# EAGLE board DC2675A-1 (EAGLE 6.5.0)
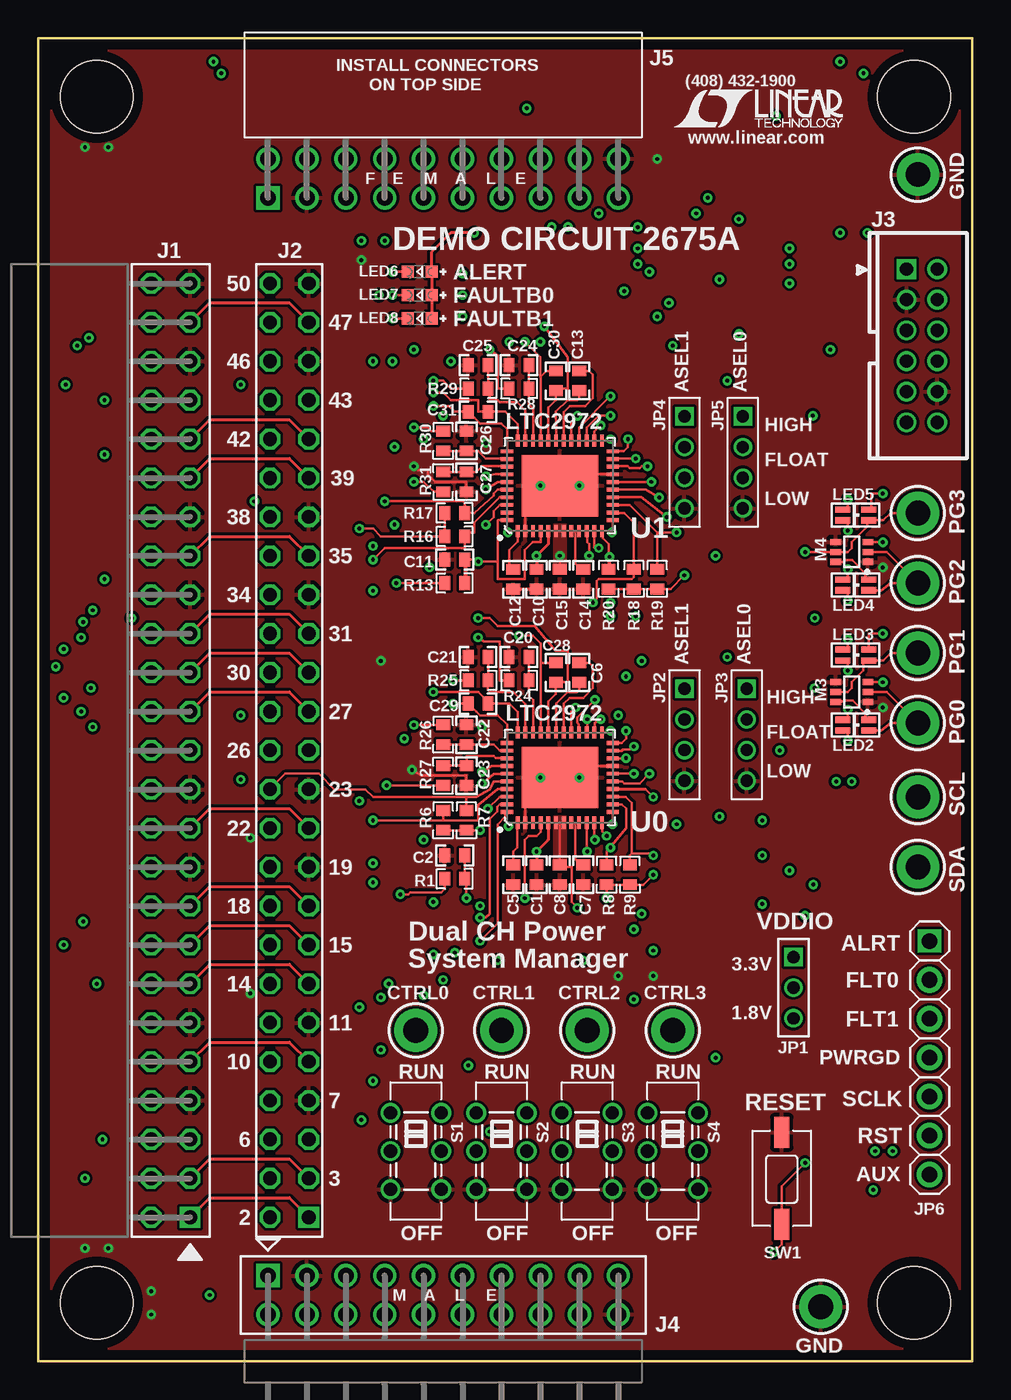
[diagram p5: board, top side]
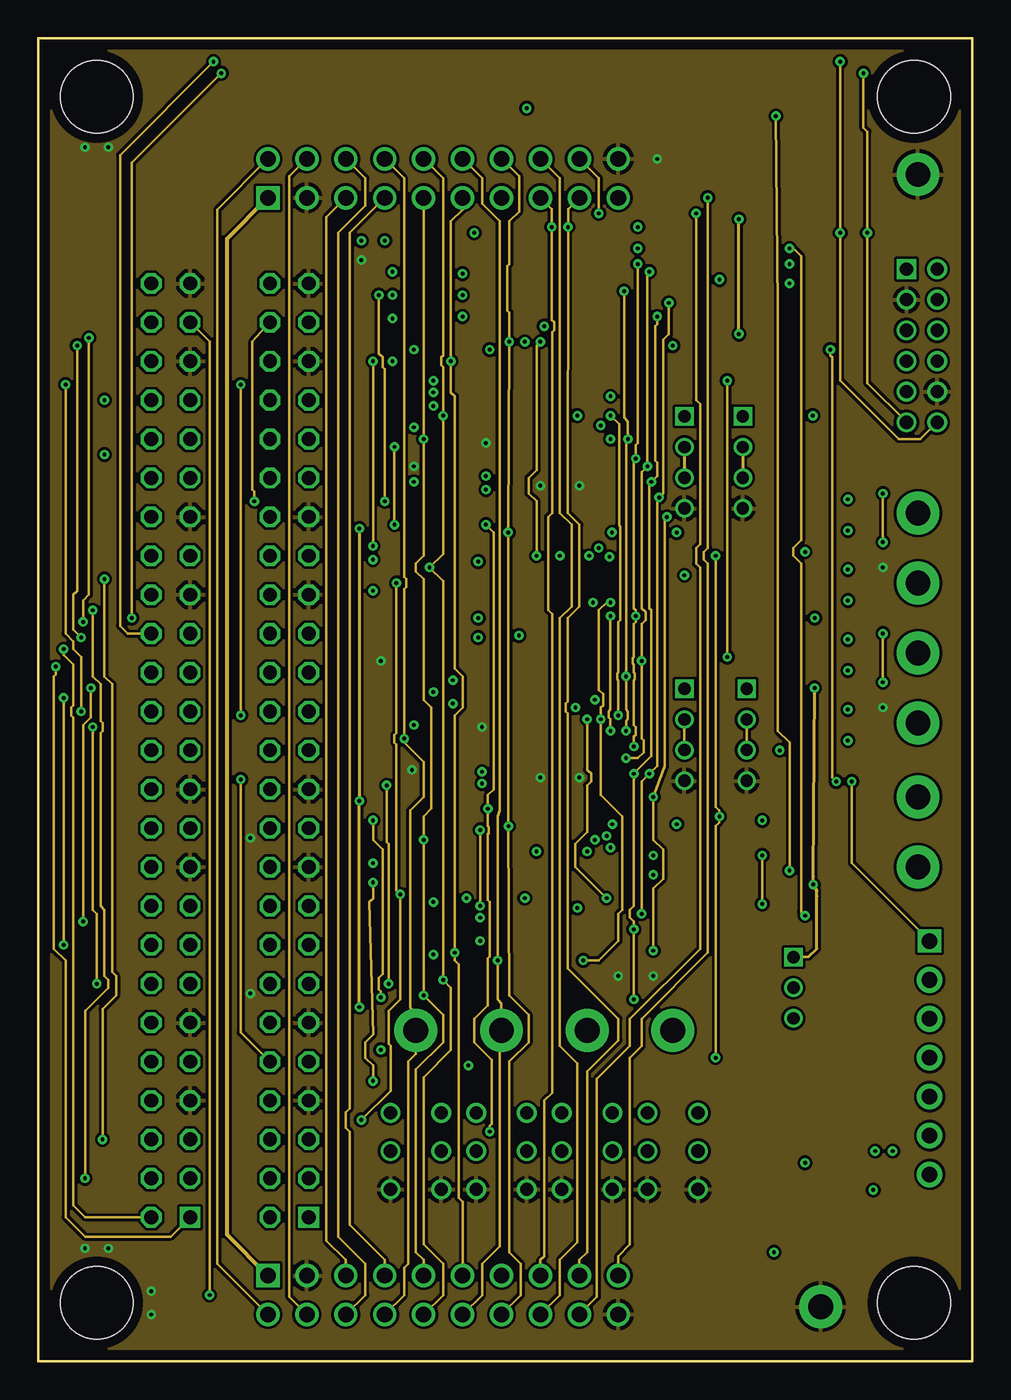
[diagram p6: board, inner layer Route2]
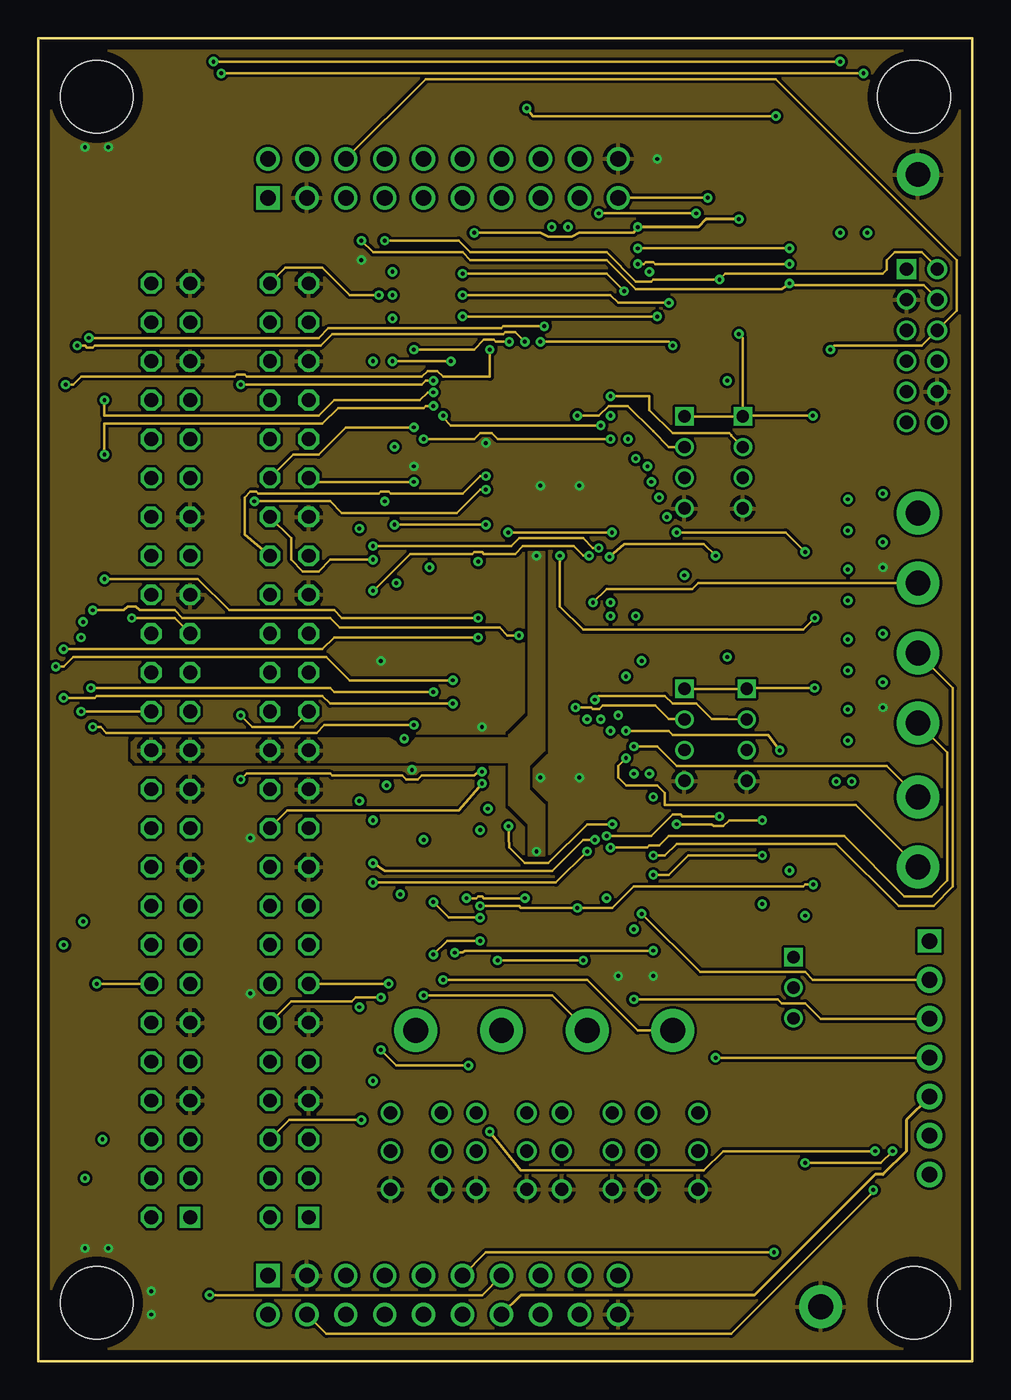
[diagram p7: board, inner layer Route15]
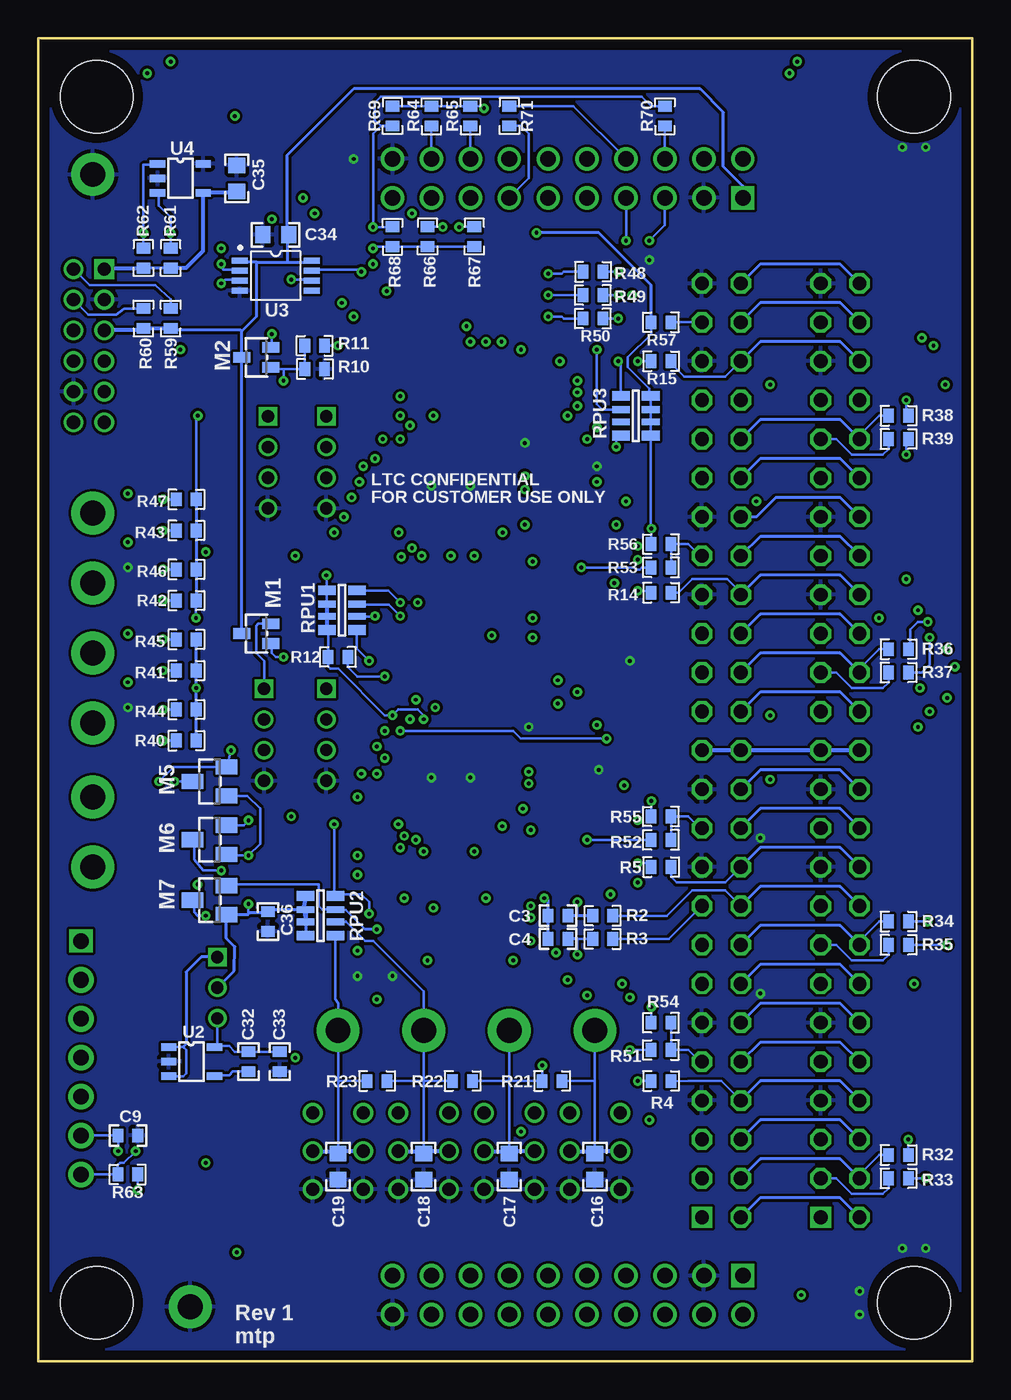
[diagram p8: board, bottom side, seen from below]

Size 60.96 x 86.36 mm. Coordinates in mm from the lower left corner, seen from the top.
Outline: 0,0 0,86.36 60.96,86.36 60.96,0 0.13,0
Copper layers (1*2+15*16): Top 0.07mm / dielectric 0.2mm / Route2 0.035mm / dielectric 1mm / Route15 0.035mm / dielectric 0.2mm / Bottom 0.07mm
Design rules "default *": minimum track width 6mil, minimum drill 10mil, track to track 6mil, track to pad 6mil, pad to pad 6mil, via to via 6mil, smd to smd 4mil, copper to edge 25mil, drill to drill 15mil, minimum pad ring 7mil, minimum via ring 7mil, stop-mask expansion 4mil, vias tented up to drill 15mil, thermal gap 10mil
Holes 4.75 mm at 3.81,3.81 3.81,82.55 57.15,82.55 57.15,3.81

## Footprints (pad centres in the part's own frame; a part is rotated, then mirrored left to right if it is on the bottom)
C0402_BOX = smd 0.7 x 0.9: 1 -0.65,0; 2 0.65,0
C0603_BOX = smd 1 x 1.1: 1 -0.85,0; 2 0.85,0
PINHEAD_2X25_RECEPT = drill 0.9 square: 1 1.27,-30.48 | drill 0.9 octagon: 2 -1.27,-30.48; 3 1.27,-27.94; 4 -1.27,-27.94; 5 1.27,-25.4; 6 -1.27,-25.4; 7 1.27,-22.86; 8 -1.27,-22.86; 9 1.27,-20.32; 10 -1.27,-20.32; 11 1.27,-17.78; 12 -1.27,-17.78; 13 1.27,-15.24; 14 -1.27,-15.24; 15 1.27,-12.7; 16 -1.27,-12.7; 17 1.27,-10.16; 18 -1.27,-10.16; 19 1.27,-7.62; 20 -1.27,-7.62; 21 1.27,-5.08; 22 -1.27,-5.08; 23 1.27,-2.54; 24 -1.27,-2.54; 25 1.27,0; 26 -1.27,0; 27 1.27,2.54; 28 -1.27,2.54; 29 1.27,5.08; 30 -1.27,5.08; 31 1.27,7.62; 32 -1.27,7.62; 33 1.27,10.16; 34 -1.27,10.16; 35 1.27,12.7; 36 -1.27,12.7; 37 1.27,15.24; 38 -1.27,15.24; 39 1.27,17.78; 40 -1.27,17.78; 41 1.27,20.32; 42 -1.27,20.32; 43 1.27,22.86; 44 -1.27,22.86; 45 1.27,25.4; 46 -1.27,25.4; 47 1.27,27.94; 48 -1.27,27.94; 49 1.27,30.48; 50 -1.27,30.48
PINHEAD_2X25_RECEPT_NO_SILK = drill 0.9 square: 1 1.27,-30.48 | drill 0.9 octagon: 2 -1.27,-30.48; 3 1.27,-27.94; 4 -1.27,-27.94; 5 1.27,-25.4; 6 -1.27,-25.4; 7 1.27,-22.86; 8 -1.27,-22.86; 9 1.27,-20.32; 10 -1.27,-20.32; 11 1.27,-17.78; 12 -1.27,-17.78; 13 1.27,-15.24; 14 -1.27,-15.24; 15 1.27,-12.7; 16 -1.27,-12.7; 17 1.27,-10.16; 18 -1.27,-10.16; 19 1.27,-7.62; 20 -1.27,-7.62; 21 1.27,-5.08; 22 -1.27,-5.08; 23 1.27,-2.54; 24 -1.27,-2.54; 25 1.27,0; 26 -1.27,0; 27 1.27,2.54; 28 -1.27,2.54; 29 1.27,5.08; 30 -1.27,5.08; 31 1.27,7.62; 32 -1.27,7.62; 33 1.27,10.16; 34 -1.27,10.16; 35 1.27,12.7; 36 -1.27,12.7; 37 1.27,15.24; 38 -1.27,15.24; 39 1.27,17.78; 40 -1.27,17.78; 41 1.27,20.32; 42 -1.27,20.32; 43 1.27,22.86; 44 -1.27,22.86; 45 1.27,25.4; 46 -1.27,25.4; 47 1.27,27.94; 48 -1.27,27.94; 49 1.27,30.48; 50 -1.27,30.48
CONN_DC1613 = drill 0.86 square: 1 -5,-1 | drill 0.86: 2 -5,1; 3 -3,-1; 4 -3,1; 5 -1,-1; 6 -1,1; 7 1,-1; 8 1,1; 9 3,-1; 10 3,1; 11 5,-1; 12 5,1
HEADER_2X10_0.1INCH = drill 1.016 square: P$1 1.27,11.43 | drill 1.016: P$2 -1.27,11.43; P$3 1.27,8.89; P$4 -1.27,8.89; P$5 1.27,6.35; P$6 -1.27,6.35; P$7 1.27,3.81; P$8 -1.27,3.81; P$9 1.27,1.27; P$10 -1.27,1.27; P$11 1.27,-1.27; P$12 -1.27,-1.27; P$13 1.27,-3.81; P$14 -1.27,-3.81; P$15 1.27,-6.35; P$16 -1.27,-6.35; P$17 1.27,-8.89; P$18 -1.27,-8.89; P$19 1.27,-11.43; P$20 -1.27,-11.43
RECEPT_2X10_0.1INCH = drill 1.016 square: P$1 -1.27,11.43 | drill 1.016: P$2 1.27,11.43; P$3 -1.27,8.89; P$4 1.27,8.89; P$5 -1.27,6.35; P$6 1.27,6.35; P$7 -1.27,3.81; P$8 1.27,3.81; P$9 -1.27,1.27; P$10 1.27,1.27; P$11 -1.27,-1.27; P$12 1.27,-1.27; P$13 -1.27,-3.81; P$14 1.27,-3.81; P$15 -1.27,-6.35; P$16 1.27,-6.35; P$17 -1.27,-8.89; P$18 1.27,-8.89; P$19 -1.27,-11.43; P$20 1.27,-11.43
1X03-2MM = drill 0.8 square: 1 -2,0 | drill 0.8: 2 0,0; 3 2,0
1X04-2MM = drill 0.8 square: 1 -3,0 | drill 0.8: 2 -1,0; 3 1,0; 4 3,0
1X07 = drill 1.016 square: 1 -7.62,0 | drill 1.016 pad 1.676: 2 -5.08,0; 3 -2.54,0; 4 0,0; 5 2.54,0; 6 5.08,0; 7 7.62,0
LED-DUAL_1.6X0.8MM = smd 1 x 0.4: 1 0.85,-0.35; 2 -0.85,-0.35; 3 0.85,0.35; 4 -0.85,0.35
CHIPLED_0603 = smd 0.8 x 0.8: N 0,0.78; P 0,-0.78
SOT323 = smd 0.7 x 1.1: 1 -0.65,-0.95; 2 0.65,-0.95; 3 0,0.95
SOT-363 = smd 0.7 x 0.4: 1 -1.05,0.65; 2 -1.05,0; 3 -1.05,-0.65; 4 1.05,-0.65; 5 1.05,0; 6 1.05,0.65
SOT23 = smd 1 x 1.4: 1 -0.95,-1.1; 2 0.95,-1.1; 3 0,1.1
R0402_BOX = smd 0.7 x 0.9: 1 -0.65,0; 2 0.65,0
R_VISHAY_CRA06S = smd 1.15 x 0.63: R1_1 -0.975,1.295; R1_2 0.975,1.295; R4_1 -0.975,-1.295; R4_2 0.975,-1.295 | smd 1.15 x 0.44: R2_1 -0.975,0.4; R2_2 0.975,0.4; R3_1 -0.975,-0.4; R3_2 0.975,-0.4
JS202011CQN = drill 0.86: 1 -2.5,1.65; 2 0,1.65; 3 2.5,1.65; 4 -2.5,-1.65; 5 0,-1.65; 6 2.5,-1.65
SWITCH_PTS635 = smd 2 x 1: SW1 -3,0; SW2 3,0
TURRET_SMALL_2308 = drill 1.626 pad 2.794: TP1 0,0
QFN44-6X7 = smd 0.8 x 0.25: 1 -2.95,2.75; 2 -2.95,2.25; 3 -2.95,1.75; 4 -2.95,1.25; 5 -2.95,0.75; 6 -2.95,0.25; 7 -2.95,-0.25; 8 -2.95,-0.75; 9 -2.95,-1.25; 10 -2.95,-1.75; 11 -2.95,-2.25; 12 -2.95,-2.75; 23 2.95,-2.75; 24 2.95,-2.25; 25 2.95,-1.75; 26 2.95,-1.25; 27 2.95,-0.75; 28 2.95,-0.25; 29 2.95,0.25; 30 2.95,0.75; 31 2.95,1.25; 32 2.95,1.75; 33 2.95,2.25; 34 2.95,2.75 | smd 0.25 x 0.8: 13 -2.25,-3.45; 14 -1.75,-3.45; 15 -1.25,-3.45; 16 -0.75,-3.45; 17 -0.25,-3.45; 18 0.25,-3.45; 19 0.75,-3.45; 20 1.25,-3.45; 21 1.75,-3.45; 22 2.25,-3.45; 35 2.25,3.45; 36 1.75,3.45; 37 1.25,3.45; 38 0.75,3.45; 39 0.25,3.45; 40 -0.25,3.45; 41 -0.75,3.45; 42 -1.25,3.45; 43 -1.75,3.45; 44 -2.25,3.45 | smd 4 x 5: 45 0,0
SOT-23-5 = smd 1 x 0.5: 1 -1.649,0.95; 2 -1.649,0; 3 -1.649,-0.95; 4 1.333,-0.95; 5 1.333,0.95
MSOP-8 = smd 0.406 x 1.016: 1 -0.975,-2.35; 2 -0.325,-2.35; 3 0.325,-2.35; 4 0.975,-2.35; 5 0.975,2.35; 6 0.325,2.35; 7 -0.325,2.35; 8 -0.975,2.35
SOT-23-5' = smd 1 x 0.5: 1 -1.491,0.95; 2 -1.491,0; 3 -1.491,-0.95; 4 1.491,-0.95; 5 1.491,0.95

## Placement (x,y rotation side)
C1  0.1uF/16V  [C0402_BOX]  32.51,31.75 270 top
C2  0.1uF/16V  [C0402_BOX]  27.18,33.02 0 top
C3  1uF/16V  [C0402_BOX]  27.05,29.08 0 bottom
C4  1uF/16V  [C0402_BOX]  27.05,27.56 0 bottom
C5  10nF  [C0402_BOX]  30.99,31.75 90 top
C6  0.1uF  [C0402_BOX]  35.31,44.96 270 top
C7  0.1uF  [C0402_BOX]  35.56,31.75 270 top
C8  0.1uF  [C0402_BOX]  34.04,31.75 270 top
C9  10n  [C0402_BOX]  55.12,14.73 180 bottom
C10  0.1uF/16V  [C0402_BOX]  32.51,51.05 270 top
C11  0.1uF/16V  [C0402_BOX]  27.18,52.32 0 top
C12  10nF  [C0402_BOX]  30.99,51.05 90 top
C13  0.1uF  [C0402_BOX]  35.31,64.01 270 top
C14  0.1uF  [C0402_BOX]  35.56,51.05 270 top
C15  0.1uF  [C0402_BOX]  34.04,51.05 270 top
C16  1uF  [C0603_BOX]  24.64,12.7 270 bottom
C17  1uF  [C0603_BOX]  30.23,12.7 270 bottom
C18  1uF  [C0603_BOX]  35.81,12.7 270 bottom
C19  1uF  [C0603_BOX]  41.4,12.7 270 bottom
C20  10n  [C0402_BOX]  31.37,45.97 180 top
C21  10n  [C0402_BOX]  28.7,45.97 180 top
C22  10n  [C0402_BOX]  27.94,40.89 90 top
C23  10n  [C0402_BOX]  27.94,38.23 270 top
C24  10n  [C0402_BOX]  31.37,65.02 180 top
C25  10n  [C0402_BOX]  28.7,65.02 180 top
C26  10n  [C0402_BOX]  27.94,60.07 90 top
C27  10n  [C0402_BOX]  27.94,57.4 270 top
C28  10n  [C0402_BOX]  33.78,44.96 90 top
C29  10n  [C0402_BOX]  28.7,42.93 180 top
C30  10n  [C0402_BOX]  33.78,64.01 90 top
C31  10n  [C0402_BOX]  28.7,61.98 180 top
C32  10nF  [C0402_BOX]  47.24,19.56 270 bottom
C33  4.7uF/10V  [C0402_BOX]  45.21,19.56 270 bottom
C34  1uF  [C0603_BOX]  45.47,73.53 180 bottom
C35  1uF  [C0603_BOX]  48.01,77.22 90 bottom
C36  0.1uF  [C0402_BOX]  45.97,28.7 270 bottom
DRILEGEND  [DRILEGEND]  not placed on the board
J1  CONN_2X25_RECEPT  [PINHEAD_2X25_RECEPT]  8.64,39.88 0 top
J2  CONN_2X25_RECEPT_NO_SILK  [PINHEAD_2X25_RECEPT_NO_SILK]  16.38,39.88 0 top
J3  CONN_DC1613  [CONN_DC1613]  57.66,66.29 270 top
J4  HEADER_CONN_2X10_0.1INCH  [HEADER_2X10_0.1INCH]  26.42,4.32 90 top
J5  RECEPT_CONN_2X10_0.1INCH  [RECEPT_2X10_0.1INCH]  26.42,77.22 90 top
JP1  [1X03-2MM]  49.28,24.38 270 top
JP2  [1X04-2MM]  42.16,40.89 270 top
JP3  [1X04-2MM]  46.23,40.89 270 top
JP4  [1X04-2MM]  42.16,58.67 270 top
JP5  [1X04-2MM]  45.97,58.67 270 top
JP6  [1X07]  58.17,19.81 270 top
LED2  Kingbright  [LED-DUAL_1.6X0.8MM]  53.34,41.53 180 top
LED3  Kingbright  [LED-DUAL_1.6X0.8MM]  53.34,46.1 180 top
LED4  Kingbright  [LED-DUAL_1.6X0.8MM]  53.34,50.67 180 top
LED5  Kingbright  [LED-DUAL_1.6X0.8MM]  53.34,55.24 180 top
LED6  RED  [CHIPLED_0603]  24.89,71.12 90 top
LED7  RED  [CHIPLED_0603]  24.89,69.6 90 top
LED8  RED  [CHIPLED_0603]  24.89,68.07 90 top
M1  NTS4173P  [SOT323]  46.74,47.5 90 bottom
M2  NTS4173P  [SOT323]  46.74,65.53 90 bottom
M3  [SOT-363]  53.09,43.69 180 top
M4  [SOT-363]  53.09,52.83 180 top
M5  BSS138  [SOT23]  49.78,37.85 90 bottom
M6  BSS138  [SOT23]  49.78,34.04 90 bottom
M7  BSS138  [SOT23]  49.78,30.1 90 bottom
R1  0  [R0402_BOX]  27.18,31.5 180 top
R2  0  [R0402_BOX]  24.13,29.08 180 bottom
R3  0  [R0402_BOX]  24.13,27.56 180 bottom
R4  0  [R0402_BOX]  20.32,18.29 0 bottom
R5  0  [R0402_BOX]  20.32,32.26 0 bottom
R6  10k  [R0402_BOX]  26.42,35.31 270 top
R7  10k  [R0402_BOX]  27.94,35.31 270 top
R8  10k  [R0402_BOX]  37.08,31.75 270 top
R9  10k  [R0402_BOX]  38.61,31.75 270 top
R10  150k  [R0402_BOX]  42.93,64.77 0 bottom
R11  49.9k  [R0402_BOX]  42.93,66.29 180 bottom
R12  10k  [R0402_BOX]  41.4,45.97 180 bottom
R13  0  [R0402_BOX]  27.18,50.8 180 top
R14  0  [R0402_BOX]  20.32,50.16 0 bottom
R15  0  [R0402_BOX]  20.32,65.28 0 bottom
R16  10k  [R0402_BOX]  27.18,53.85 180 top
R17  10k  [R0402_BOX]  27.18,55.37 180 top
R18  10k  [R0402_BOX]  38.86,51.05 270 top
R19  10k  [R0402_BOX]  40.39,51.05 270 top
R20  10k  [R0402_BOX]  37.21,51.05 270 top
R21  0  [R0402_BOX]  27.43,18.29 0 bottom
R22  0  [R0402_BOX]  33.27,18.29 0 bottom
R23  0  [R0402_BOX]  38.86,18.29 0 bottom
R24  0  [R0402_BOX]  31.37,44.45 0 top
R25  0  [R0402_BOX]  28.7,44.45 0 top
R26  0  [R0402_BOX]  26.42,40.89 270 top
R27  0  [R0402_BOX]  26.42,38.23 90 top
R28  0  [R0402_BOX]  31.37,63.5 0 top
R29  0  [R0402_BOX]  28.7,63.5 0 top
R30  0  [R0402_BOX]  26.42,60.07 270 top
R31  0  [R0402_BOX]  26.42,57.4 90 top
R32  0  [R0402_BOX]  4.83,13.46 0 bottom
R33  0  [R0402_BOX]  4.83,11.94 0 bottom
R34  0  [R0402_BOX]  4.83,28.7 0 bottom
R35  0  [R0402_BOX]  4.83,27.18 0 bottom
R36  0  [R0402_BOX]  4.83,46.48 0 bottom
R37  0  [R0402_BOX]  4.83,44.96 0 bottom
R38  0  [R0402_BOX]  4.83,61.72 0 bottom
R39  0  [R0402_BOX]  4.83,60.2 0 bottom
R40  1.4k  [R0402_BOX]  51.31,40.51 0 bottom
R41  1.4k  [R0402_BOX]  51.31,45.09 0 bottom
R42  1.4k  [R0402_BOX]  51.31,49.66 0 bottom
R43  1.4k  [R0402_BOX]  51.31,54.23 0 bottom
R44  4k  [R0402_BOX]  51.31,42.55 0 bottom
R45  4k  [R0402_BOX]  51.31,47.12 0 bottom
R46  4k  [R0402_BOX]  51.31,51.69 0 bottom
R47  4k  [R0402_BOX]  51.31,56.26 0 bottom
R48  866  [R0402_BOX]  24.77,71.12 0 bottom
R49  866  [R0402_BOX]  24.77,69.6 180 bottom
R50  866  [R0402_BOX]  24.77,68.07 180 bottom
R51  0  [R0402_BOX]  20.32,20.32 180 bottom
R52  0  [R0402_BOX]  20.32,34.04 180 bottom
R53  0  [R0402_BOX]  20.32,51.82 180 bottom
R54  10k  [R0402_BOX]  20.32,22.1 180 bottom
R55  10k  [R0402_BOX]  20.32,35.56 180 bottom
R56  10k  [R0402_BOX]  20.32,53.34 180 bottom
R57  10k  [R0402_BOX]  20.32,67.82 180 bottom
R59  10k  [R0402_BOX]  52.32,68.07 90 bottom
R60  10k  [R0402_BOX]  54.1,68.07 90 bottom
R61  10k  [R0402_BOX]  52.32,72.01 270 bottom
R62  10k  [R0402_BOX]  54.1,72.01 270 bottom
R63  0 (DNI)  [R0402_BOX]  55.12,12.19 180 bottom
R64  0  [R0402_BOX]  35.31,81.28 90 bottom
R65  0  [R0402_BOX]  32.77,81.28 90 bottom
R66  0  [R0402_BOX]  35.56,73.41 270 bottom
R67  0  [R0402_BOX]  32.51,73.41 270 bottom
R68  10k  [R0402_BOX]  37.85,73.41 90 bottom
R69  10k  [R0402_BOX]  37.85,81.28 270 bottom
R70  10k  [R0402_BOX]  20.07,81.28 90 bottom
R71  0 (DNI)  [R0402_BOX]  30.23,81.28 270 bottom
RPU1  10k, 4X  [R_VISHAY_CRA06S]  41.15,49.02 180 bottom
RPU2  10k, 4X  [R_VISHAY_CRA06S]  42.55,29.08 180 bottom
RPU3  10k, 4X  [R_VISHAY_CRA06S]  21.97,61.72 0 bottom
S1  CONTROL0  [JS202011CQN]  24.64,13.72 270 top
S2  CONTROL1  [JS202011CQN]  30.23,13.72 270 top
S3  CONTROL2  [JS202011CQN]  35.81,13.72 270 top
S4  CONTROL3  [JS202011CQN]  41.4,13.72 270 top
SW1  PTS635SL25SMTR LFS  [SWITCH_PTS635]  48.51,11.94 90 top
TP1  [TURRET_SMALL_2308]  57.4,36.83 0 top
TP2  [TURRET_SMALL_2308]  57.4,32.26 0 top
TP3  [TURRET_SMALL_2308]  57.4,41.66 0 top
TP4  [TURRET_SMALL_2308]  57.4,46.23 0 top
TP5  [TURRET_SMALL_2308]  57.4,50.8 0 top
TP6  [TURRET_SMALL_2308]  57.4,55.37 0 top
TP7  [TURRET_SMALL_2308]  24.64,21.59 0 top
TP8  [TURRET_SMALL_2308]  30.23,21.59 0 top
TP9  [TURRET_SMALL_2308]  35.81,21.59 0 top
TP10  [TURRET_SMALL_2308]  41.4,21.59 0 top
TP11  [TURRET_SMALL_2308]  57.4,77.47 0 top
TP12  [TURRET_SMALL_2308]  51.05,3.56 0 top
U0  LTC2972  [QFN44-6X7]  34.04,38.1 90 top
U1  LTC2972  [QFN44-6X7]  34.04,57.15 90 top
U2  LT1761-1.8V  [SOT-23-5]  50.8,19.56 0 bottom
U3  LTC4313-3  [MSOP-8]  45.47,70.87 270 bottom
U4  24AA02T-I/OT  [SOT-23-5']  51.69,77.22 0 bottom
U$6  [DC2675_FRAME]  not placed on the board
U$86  [LT_LOGO_SILK_450MILS]  41.4,80.52 0 top

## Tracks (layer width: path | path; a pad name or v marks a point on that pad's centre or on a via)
1V8
  Bottom 0.152: C33.1 C32.1 48.15,20.21 48.51,20.57 49.4,20.57 U2.5 49.28,20.7 JP1.3
ALERTB  (via drill 0.25)
  Top 0.152: U1.22 38.19,59.4 38.48,59.69 v38.48,60.2 | U0.22 38.06,40.35 38.35,40.64 v38.35,41.15
  Route2 0.152: v38.23,69.85 38.23,61.59 38.48,61.34 v38.48,60.2 38.35,59.94 v38.35,44.7 38.35,42.55 38.48,42.42 38.48,41.91 38.35,41.78 v38.35,41.15 | v53.09,37.85 53.09,32.51 JP6.1
  Route15 0.152: v38.23,69.85 37.08,70.99 v27.69,70.99 | v38.35,41.15 41.15,41.15 41.4,40.89 47.62,40.89 v48.39,39.88
  Bottom 0.152: R12.1 40.75,45.32 40.13,44.7 v38.35,44.7 | v48.39,39.88 48.64,38.84 M5.2 52.14,38.8 v53.09,37.85 | R48.1 26.67,71.12 26.8,70.99 v27.69,70.99
ALERTB_3V3  (via drill 0.25)
  Route2 0.152: J4.P$6 21.34,4.32 21.34,6.35 19.56,8.13 19.56,73.66 21.34,75.44 21.34,77.22 J5.P$6 | v51.69,66.04 51.69,65.66 51.82,65.53 51.82,38.1 v52.07,37.85
  Route15 0.152: J5.P$6 25.27,83.69 48.13,83.69 59.94,71.88 59.94,68.58 J3.6 57.66,66.29 51.94,66.29 v51.69,66.04
  Bottom 0.152: R70.1 J5.P$6 | v52.07,37.85 M5.3
ASEL0_U0  (via drill 0.25)
  Top 0.152: U0.26 35.28,41.58 35.18,41.68 35.18,42.04 v36.32,43.18
  Route2 0.152: JP3.2 JP3.3
  Route15 0.152: v36.32,43.18 36.58,43.43 40.89,43.43 41.4,42.93 42.93,42.93 43.94,41.91 44.94,41.91 JP3.2
ASEL0_U1  (via drill 0.25)
  Top 0.152: U1.26 35.29,60.94 v37.34,62.99
  Route2 0.203: JP5.2 JP5.3
  Route15 0.152: v37.34,62.99 39.88,62.99 39.88,62.1 41.4,60.58 45.09,60.58 45.21,60.45 45.21,60.44 JP5.2
ASEL1_U0  (via drill 0.25)
  Top 0.152: U0.27 34.79,42.41 v35.05,42.67
  Route2 0.152: JP2.2 JP2.3
  Route15 0.152: v35.05,42.67 36.07,42.67 36.17,42.57 36.6,42.57 36.83,42.8 40.26,42.8 41.15,41.91 42.15,41.91 JP2.2
ASEL1_U1  (via drill 0.25)
  Top 0.152: U1.27 34.79,61.33 v35.18,61.72
  Route2 0.203: JP4.2 JP4.3
  Route15 0.152: v35.18,61.72 36.58,61.72 37.21,62.36 38.48,62.36 40.13,60.71 41.15,59.67 JP4.2
AUX_SCL  (via drill 0.25)
  Top 0.203: J1.31 11.18,48.77 16.38,48.77 J2.31
  Route2 0.152: J3.11 54.1,63.85 v54.1,73.66 54.1,80.26 53.85,80.52 v53.85,84.07 | v11.94,84.07 6.1,78.23 v6.1,48.51
  Route15 0.152: v53.85,84.07 v11.94,84.07 | v6.1,48.51 8.89,48.51 J1.31
  Bottom 0.152: U4.1 53.24,78.11 54.1,78.11 v54.1,73.66 R62.1
AUX_SDA  (via drill 0.25)
  Route2 0.152: J3.12 57.56,60.2 56.13,60.2 52.32,64.01 v52.32,73.66 v52.32,84.84 | v11.43,84.84 5.33,78.74 5.33,48.01 5.84,47.5 J1.32
  Route15 0.152: v52.32,84.84 v11.43,84.84
  Bottom 0.152: U4.3 53.09,76.17 53.09,75.44 52.32,74.68 v52.32,73.66 R61.1
  Bottom 0.203: J1.32 8.64,48.77 13.84,48.77 J2.32
AUXFAULTB  (via drill 0.25)
  Top 0.152: U0.42 30.57,36.83 30.1,36.83 v29.34,36.07 | U1.42 30.12,55.9 29.72,55.5 29.72,55.12 v29.21,54.61
  Route2 0.152: v29.46,14.99 29.46,15.37 29.59,15.49 29.59,19.68 28.45,20.83 28.45,22.35 29.34,23.24 29.34,26.29 29.46,26.42 29.46,29.97 29.34,30.1 29.34,34.42 29.39,34.47 29.39,34.87 29.34,34.92 v29.34,36.07 29.34,36.96 29.72,37.34 29.72,54.1 v29.21,54.61 | v23.24,54.61 v23.24,59.69
  Route15 0.152: v54.61,13.72 44.7,13.72 43.43,12.45 31.5,12.45 v29.46,14.99 | v29.21,54.61 v23.24,54.61
  Bottom 0.152: JP6.7 R63.2 55.77,12.81 55.63,12.95 55.37,12.95 v54.61,13.72 | v23.24,59.69 23.24,60.13 RPU3.R4_1
AUXFAULTB_3V3  (via drill 0.25)
  Route2 0.152: J4.P$4 16.38,4.19 16.38,77.34 J5.P$4
  Route15 0.152: v54.48,11.18 54.48,11.05 45.21,1.78 18.8,1.78 J4.P$4
  Bottom 0.152: R63.1 54.47,11.19 v54.48,11.18
CTRL0  (via drill 0.25)
  Top 0.152: U0.23 37.24,41.05 v37.34,41.15
  Route2 0.152: J4.P$8 23.88,4.32 23.88,6.1 24.13,6.35 24.13,19.56 24.64,20.07 TP7.TP1 24.64,22.35 24.26,23.11 24.26,35.94 25.15,36.83 25.15,39.12 23.88,40.39 v23.88,40.64 23.88,50.42 24,50.55 24,51.05 23.88,51.18 23.88,77.22 J5.P$8 | v37.34,41.15 37.34,41.91 37.24,42.04 37.24,42.42 37.34,42.55 v37.34,48.64
  Bottom 0.152: R21.2 24.64,18.29 | 24.64,18.29 C16.1 | 24.64,18.29 TP7.TP1 | v37.34,41.15 29.97,41.15 29.46,40.64 v23.88,40.64 | v37.34,48.64 38.1,49.4 40.15,49.4 RPU1.R3_1 | R71.1 26.05,81.93 J5.P$8
  Bottom 0.254: S1.5 24.64,13.72 | S1.2 24.64,13.72 | 24.64,13.72 C16.1
CTRL1  (via drill 0.25)
  Top 0.152: 36.32,41.4 36.32,41.09 U0.24 36.29,41.37 36.32,41.4 | 36.32,41.4 36.32,41.66 v36.7,41.91
  Route2 0.152: J4.P$12 28.96,4.32 28.96,6.35 30.1,7.49 30.1,20.07 30.23,21.08 TP8.TP1 30.23,23.37 29.97,23.62 v29.97,26.16 29.97,35.56 30.1,35.94 30.1,74.42 28.96,75.56 28.96,77.22 J5.P$12 | v37.34,49.53 37.08,49.53 36.58,49.02 36.58,43.81 36.85,43.56 36.85,42.8 36.7,42.67 v36.7,41.91 36.7,36.96 38.1,35.56 38.1,29.46 37.85,29.21 37.85,27.43 36.58,26.16 v35.56,26.16
  Route15 0.152: v22.35,20.32 23.37,19.3 v28.07,19.3 | v35.56,26.16 v29.97,26.16
  Bottom 0.152: 30.23,18.29 R21.1 28.07,18.3 v28.07,19.3 | 30.23,18.29 C17.1 | R22.2 30.23,18.29 | 30.23,18.29 TP8.TP1 | RPU1.R4_1 38.12,50.32 v37.34,49.53 | R51.2 v22.35,20.32
  Bottom 0.254: S2.5 30.23,13.72 | S2.2 30.23,13.72 | 30.23,13.72 C17.1
CTRL2  (via drill 0.25)
  Top 0.152: U1.23 37.24,60.1 v37.34,60.2
  Route2 0.152: J4.P$9 25.15,6.6 24.64,7.11 24.64,19.05 26.42,20.83 26.42,22.61 v25.15,23.88 v25.15,34.04 25.15,35.56 25.65,36.07 25.65,42.67 25.15,43.18 25.15,51.05 24.64,51.56 24.64,52.07 25.15,52.58 v25.15,60.2 J5.P$9
  Route15 0.152: v37.34,60.2 29.97,60.2 29.59,60.58 28.83,60.58 28.45,60.2 v25.15,60.2 | TP9.TP1 33.53,23.88 v25.15,23.88
  Bottom 0.152: R22.1 35.81,18.29 | 35.81,18.29 C18.1 | R23.2 35.81,18.29 | 35.81,18.29 TP9.TP1 35.81,24.13 39.12,27.43 39.62,27.43 40.89,28.7 40.91,28.68 RPU2.R2_1 | R52.2 v25.15,34.04
  Bottom 0.254: S3.5 35.81,13.72 | S3.2 35.81,13.72 | 35.81,13.72 C18.1
CTRL3  (via drill 0.25)
  Top 0.152: U1.24 36.29,60.67 v36.7,61.09
  Route2 0.152: J5.P$10 26.42,77.22 26.42,65.66 26.29,65.53 26.29,65.02 26.42,64.9 v26.42,61.72 26.42,52.7 v25.53,51.82 26.42,50.93 v26.42,24.89 26.92,24.38 26.92,20.32 25.15,18.54 25.15,7.62 26.42,6.35 26.42,4.32 J4.P$10
  Route15 0.152: v36.7,61.09 26.92,61.09 26.42,61.59 v26.42,61.72 | TP10.TP1 39.12,21.59 35.81,24.89 v26.42,24.89
  Bottom 0.152: R23.1 41.4,18.29 | 41.4,18.29 C19.1 | 41.4,18.29 TP10.TP1 41.4,23.37 41.57,23.66 RPU2.R1_1 | R53.2 21.59,51.82 21.72,51.69 21.97,51.69 22.1,51.82 v25.53,51.82
  Bottom 0.254: S4.5 41.4,13.72 | S4.2 41.4,13.72 | 41.4,13.72 C19.1
DAC_CH0  (via drill 0.25)
  Top 0.152: U0.38 29.58,38.85 v28.96,38.48
  Route2 0.152: v13.21,37.97 13.21,21.46 J2.10
  Route15 0.152: v28.96,38.48 28.7,38.48 28.45,38.23 25.02,38.23 24.77,37.97 24,37.97 23.75,38.23 19.18,38.23 19.05,38.35 13.59,38.35 v13.21,37.97
  Bottom 0.203: J1.10 8.64,20.83 13.84,20.83 J2.10
DAC_CH1  (via drill 0.25)
  Top 0.152: U0.39 29.71,38.35 29.46,38.1 v28.96,37.72
  Route15 0.152: v28.96,37.72 27.43,35.94 16.26,35.94 J2.22
  Bottom 0.203: J1.22 8.64,36.07 13.84,36.07 J2.22
DAC_CH2  (via drill 0.25)
  Top 0.152: U1.38 29.83,57.9 v29.21,57.78
  Route15 0.152: v29.21,57.78 28.83,57.78 27.69,56.64 22.99,56.64 22.86,56.77 22.35,56.77 22.23,56.64 14.35,56.64 14.22,56.77 13.84,56.77 13.46,56.39 13.46,53.98 J2.36
  Bottom 0.203: J1.36 8.64,53.85 13.84,53.85 J2.36
DAC_CH3  (via drill 0.25)
  Top 0.152: U1.39 29.97,57.4 v29.21,56.9
  Route2 0.152: v14.1,56.13 14.1,56.77 13.97,56.9 13.97,66.55 J2.48
  Route15 0.152: v29.21,56.9 28.83,56.9 27.3,55.37 19.81,55.37 19.05,56.13 v14.1,56.13
  Bottom 0.203: J1.48 8.64,69.09 13.84,69.09 J2.48
FAULT1  (via drill 0.25)
  Route2 0.152: J5.P$18 36.58,77.22 v36.58,74.93 | v42.93,74.93 42.93,62.74 43.18,62.48 43.18,53.34 42.93,53.09 42.93,52.07 43.18,51.82 43.18,26.92 38.61,22.35 38.61,20.57 36.45,18.41 36.45,4.19 J4.P$18
  Route15 0.152: v36.58,74.93 v42.93,74.93
  Bottom 0.152: R64.1 J5.P$18
FAULT2
  Route2 0.152: J5.P$16 34.04,77.22 34.04,55.37 34.8,54.61 34.8,49.28 34.04,48.51 34.04,20.57 35.18,19.43 35.18,7.75 34.04,6.6 34.04,4.32 J4.P$16
  Bottom 0.152: R65.1 J5.P$16
FAULT3  (via drill 0.25)
  Route2 0.152: J4.P$17 35.31,6.6 35.81,7.11 35.81,18.92 37.85,20.95 37.85,22.35 34.54,25.65 34.54,42.29 34.42,42.42 34.42,42.93 34.54,43.05 34.54,48.51 35.31,49.28 35.31,54.61 34.54,55.37 v34.57,74.04 34.57,75.21 J5.P$17
  Bottom 0.152: R66.1 34.56,74.06 v34.57,74.04
FAULT4  (via drill 0.25)
  Route2 0.152: J4.P$15 32.77,6.6 33.02,6.86 33.02,17.02 33.53,17.53 33.53,48.77 33.27,49.02 33.27,55.12 33.53,55.37 33.53,67.18 33.66,67.31 33.66,67.82 33.5,67.97 v33.5,74.04 33.5,75.21 J5.P$15
  Bottom 0.152: R67.1 33.51,74.06 v33.5,74.04
FAULTB0  (via drill 0.25)
  Top 0.152: U0.17 38.1,37.85 38.23,37.72 39.24,37.72 v39.88,38.35 | v40.51,56.39 39.62,56.9 U1.17
  Route2 0.152: v39.37,29.21 39.37,37.85 v39.88,38.35 40.39,38.86 40.39,56.26 v40.51,56.39 40.77,56.64 40.77,66.67 41.15,67.06 v41.15,69.09
  Route15 0.152: JP6.2 50.55,24.89 50.04,25.4 43.18,25.4 v39.37,29.21 | v47.24,35.31 45.09,35.31 44.7,34.92 44.07,34.92 43.94,35.05 v41.66,35.05 | v27.69,69.6 37.34,69.6 37.85,69.09 v41.15,69.09
  Bottom 0.152: v39.37,29.21 39.37,29.97 39.88,30.48 41.59,30.48 RPU2.R4_1 41.66,30.42 v41.66,35.05 | M6.2 47.56,34.99 v47.24,35.31 | R49.2 v27.69,69.6
FAULTB1  (via drill 0.25)
  Top 0.152: U1.18 v40.01,57.4 | v38.86,38.35 U0.18
  Route2 0.152: v38.86,23.62 v38.86,28.19 38.86,28.7 38.61,28.96 38.61,29.46 38.86,29.72 v38.86,38.35 40.01,39.5 40.01,49.02 39.88,49.15 39.88,57.28 v40.01,57.4 40.39,57.78 40.39,58.67 40.26,58.8 40.26,67.56 40.39,67.69 v40.39,68.2
  Route15 0.152: v38.86,23.62 48.26,23.62 48.51,23.37 50.04,23.37 51.05,22.35 JP6.3 | v27.69,68.2 v40.39,68.2
  Bottom 0.152: 39.64,28.21 39.62,28.19 v38.86,28.19 38.88,28.21 39.64,28.21 | 40.89,29.46 41.68,29.46 RPU2.R3_1 | RPU2.R3_1 40.89,29.46 | 40.89,29.46 39.64,28.21 | RPU2.R3_1 42.44,29.48 42.67,29.72 42.67,31.11 48.62,31.11 M7.2 | R50.2 26.67,68.07 26.8,68.2 v27.69,68.2
GND  (via drill 0.25)
  Top 0.152: U1.2 31.79,56.17 v32.77,57.15 U1.45 v35.31,57.15 36.06,57.9 U1.19 | U0.19 36.06,38.85 v35.31,38.1 U0.45 v32.77,38.1 31.79,37.12 U0.2 | C12.1 C10.2 | C27.2 27.94,57.4 25.91,57.4 25.4,57.91 25.4,58.17 24.77,58.17 v24.51,58.42 | C23.2 27.94,38.23 25.02,38.23 v24.38,38.61
  other vias: 29.21,59.94 55.12,51.82 55.12,42.67 28.96,41.4 40.39,78.49 40.13,25.15 13.84,24 13.84,34.16 37.85,25.15 3.05,7.37 4.57,7.37 7.37,4.57 7.37,3.05 3.05,79.25 4.57,79.25 22.35,45.72 21.08,71.88
  pour Top (isolate 0.178, rank 2): 60.2,0.76 1.78,0.76 0.76,1.65 0.76,85.6 60.2,85.6
  pour Route2 (isolate 0.178): 0.76,85.6 0.76,2.54 2.67,0.76 60.2,0.76 60.2,85.6
  pour Bottom (isolate 0.178): 60.2,0.76 60.2,85.6 0.76,85.6 0.76,1.27 1.27,0.76
  pour Route15 (isolate 0.178, rank 2): 0.76,85.6 0.76,2.03 2.16,0.76 60.2,0.76 60.2,85.6
IIN_SNSM
  Top 0.203: J1.17 11.18,30.99 16.38,30.99 J2.17
  Bottom 0.152: R3.1 19.81,27.56 J2.17
IIN_SNSP
  Bottom 0.152: R2.1 19.94,29.08 18.29,30.73 16.13,30.73 J2.18
  Bottom 0.203: J1.18 8.64,30.99 13.84,30.99 J2.18
ISM0  (via drill 0.25)
  Top 0.152: C28.2 33.77,45.59 32.81,45.59 32.79,45.61 U0.31 32.79,46.84 32.26,47.37 v31.37,47.37
  Route2 0.152: v3.56,49.02 3.56,44.7 4.06,44.2 4.06,41.78 4.19,41.66 4.19,41.15 4.06,41.02 4.06,29.72 4.32,29.46 4.32,25.15 4.57,24.89 4.57,24.38 3.05,22.86 v3.05,11.94
  Route15 0.152: v31.37,47.37 30.61,47.37 30.1,47.88 19.68,47.88 19.05,48.51 9.4,48.51 8.89,49.02 6.6,49.02 6.35,49.28 5.84,49.28 5.59,49.02 v3.56,49.02
  Bottom 0.152: v3.05,11.94 R33.2
ISM1  (via drill 0.25)
  Top 0.152: U0.35 30.59,41.55 29.97,42.16 28.83,42.16 28.57,42.42 28.18,42.8 C29.2 v27.05,42.93
  Route2 0.152: v1.65,43.31 v1.65,27.18
  Route15 0.152: v27.05,42.93 19.05,42.93 18.54,43.43 3.81,43.43 3.68,43.31 v1.65,43.31
  Bottom 0.152: v1.65,27.18 R35.2
ISM2  (via drill 0.25)
  Top 0.152: C30.2 33.77,64.64 33.15,64.64 32.79,64.28 U1.31 32.79,64.24 32.77,64.26 32.77,65.53 v31.75,66.55
  Route2 0.152: v2.54,66.29 2.54,50.29 2.29,50.04 2.29,47.75 v2.79,47.24
  Route15 0.152: v31.75,66.55 31.11,67.18 30.48,67.18 30.35,67.06 19.18,67.06 18.41,66.29 3.68,66.29 3.56,66.17 3.17,66.17 3.05,66.29 v2.54,66.29
  Bottom 0.152: v2.79,47.24 2.79,45.47 3.3,44.96 R37.2
ISM3  (via drill 0.25)
  Top 0.152: U1.35 30.59,60.85 30.23,61.21 28.83,61.21 28.45,61.59 28.18,61.85 C31.2 27.18,61.98 26.8,62.36 v25.78,62.36
  Route15 0.152: v25.78,62.36 25.27,62.36 25.15,62.23 19.56,62.23 18.54,61.21 4.32,61.21 v4.32,59.18
  Bottom 0.152: v4.32,59.18 4.32,60.06 R39.2
ISNSM_CH0
  Top 0.203: J1.3 11.18,13.21 16.38,13.21 J2.3
  Bottom 0.152: R33.1 5.48,11.29 5.84,10.92 7.87,10.92 8.89,11.94 J1.3
ISNSM_CH1
  Top 0.203: J1.15 11.18,28.45 16.38,28.45 J2.15
  Bottom 0.152: R35.1 5.48,26.53 5.84,26.16 7.87,26.16 8.89,27.18 J1.15
ISNSM_CH2
  Top 0.203: J1.29 11.18,46.23 16.38,46.23 J2.29
  Bottom 0.152: R37.1 5.48,44.31 5.84,43.94 7.87,43.94 8.89,44.96 J1.29
ISNSM_CH3
  Top 0.203: J1.41 11.18,61.47 16.38,61.47 J2.41
  Bottom 0.152: R39.1 5.48,59.55 5.84,59.18 7.87,59.18 8.89,60.2 J1.41
ISNSP_CH0
  Bottom 0.152: J1.4 7.37,12.19 6.1,13.46 R32.1
  Bottom 0.203: J1.4 8.64,13.21 13.84,13.21 J2.4
ISNSP_CH1
  Bottom 0.152: J1.16 7.37,27.43 6.1,28.7 R34.1
  Bottom 0.203: J1.16 8.64,28.45 13.84,28.45 J2.16
ISNSP_CH2
  Bottom 0.152: J1.30 7.37,45.21 6.1,46.48 R36.1
  Bottom 0.203: J1.30 8.64,46.23 13.84,46.23 J2.30
ISNSP_CH3
  Bottom 0.152: J1.42 7.37,60.45 6.1,61.72 R38.1
  Bottom 0.203: J1.42 8.64,61.47 13.84,61.47 J2.42
ISP0  (via drill 0.25)
  Top 0.152: 33.29,43.06 U0.30 33.29,42.02 33.27,42.04 33.29,43.06 | 33.29,43.06 33.78,43.56 C28.1 33.78,44.32 34.54,44.32 34.54,46.35 33.78,46.35 32.38,48.01 29.97,48.01 29.46,48.51 v28.7,48.51
  Route2 0.152: v4.32,51.05 4.32,44.7 4.83,44.2 4.83,25.4 5.08,25.15 5.08,23.88 4.19,22.99 v4.19,14.48
  Route15 0.152: v28.7,48.51 19.81,48.51 19.3,49.02 12.45,49.02 10.41,51.05 v4.32,51.05
  Bottom 0.152: v4.19,14.48 4.19,13.48 R32.2
ISP1  (via drill 0.25)
  Top 0.152: U0.34 31.29,42.37 30.73,42.93 C29.1 29.35,43.04 28.7,43.69 v25.78,43.69
  Route2 0.152: v3.43,43.94 3.43,42.04 2.92,41.53 v2.92,28.7
  Route15 0.152: v25.78,43.69 19.3,43.69 19.05,43.94 v3.43,43.94
  Bottom 0.152: v2.92,28.7 R34.2
ISP2  (via drill 0.25)
  Top 0.152: 33.29,62.24 U1.30 33.29,62.22 33.27,62.23 33.29,62.24 | 33.29,62.24 33.78,62.74 C30.1 33.78,63.5 34.54,63.5 34.54,65.53 v33.02,67.56
  Route2 0.152: v3.3,66.8 3.3,50.04 2.92,49.66 v2.92,48.26
  Route15 0.152: v33.02,67.56 30.35,67.56 30.23,67.44 18.92,67.44 18.29,66.8 v3.3,66.8
  Bottom 0.152: v2.92,48.26 3.56,48.26 4.06,47.75 4.06,46.59 R36.2
ISP3  (via drill 0.25)
  Top 0.152: U1.34 31.29,61.17 30.48,61.98 C31.1 28.7,61.98 28.7,62.74 26.92,62.74 26.42,63.25 v25.78,63.25
  Route15 0.152: v25.78,63.25 25.4,63.25 24.89,62.74 19.3,62.74 18.29,61.72 4.32,61.72 v4.32,62.74
  Bottom 0.152: v4.32,62.74 4.32,61.86 R38.2
N$1  (via drill 0.25)
  Top 0.152: U0.10 35.79,33.27 v35.81,33.27
  Route2 0.152: v21.84,31.24 21.84,30.23 21.59,29.97 21.84,21.34 21.34,20.83 21.34,19.81 21.84,19.3 v21.84,18.29
  Route15 0.152: v35.81,33.27 33.78,31.24 v21.84,31.24
  Bottom 0.152: v21.84,18.29 R4.1
N$2  (via drill 0.25)
  Top 0.152: U0.11 36.29,34.07 v36.32,34.04
  Route15 0.152: v36.32,34.04 35.56,34.04 33.53,32 22.61,32 v21.84,32.51
  Bottom 0.152: v21.84,32.51 21.22,32.51 R5.1
N$4  (via drill 0.25)
  Top 0.152: U1.10 35.81,54.17 35.81,53.47 35.94,53.34 v35.94,52.58
  Route15 0.152: v35.94,52.58 35.56,52.58 34.92,53.21 31.62,53.21 31.11,52.7 29.08,52.7 28.96,52.83 28.45,52.83 28.32,52.7 24.26,52.7 v21.84,50.29
  Bottom 0.152: v21.84,50.29 21.1,50.29 R14.1
N$5  (via drill 0.25)
  Top 0.152: U1.11 36.29,53.12 v36.58,53.09
  Route2 0.152: v21.84,53.21 v21.84,65.28
  Route15 0.152: v36.58,53.09 36.2,53.09 35.56,53.72 31.37,53.72 30.86,53.21 v21.84,53.21
  Bottom 0.152: v21.84,65.28 R15.1
N$6
  Bottom 0.152: J5.P$13 28.96,77.22 28.96,80.14 29.46,80.64 30.21,80.64 R71.2
N$8  (via drill 0.25)
  Top 0.152: v55.12,56.64 54.36,56.64 54.36,55.72 LED5.2 | v55.12,53.47 54.15,53.47 M4.3
  Route2 0.152: v55.12,56.64 v55.12,53.47
N$9
  Top 0.152: M4.6 52.45,52.17 52.59,52.28 53.13,52.28 53.98,51.44 53.98,50.93 54.19,50.93 LED4.2
N$10
  Top 0.152: M3.6 52.15,43.05 52.48,43.05 52.6,43.13 53.14,43.13 53.98,42.29 53.98,41.91 54.19,41.78 LED2.2
N$11  (via drill 0.25)
  Top 0.152: v55.12,47.5 54.19,47.5 LED3.2 | v55.12,44.32 55.12,44.34 M3.3
  Route2 0.152: v55.12,47.5 v55.12,44.32
N$12  (via drill 0.25)
  Top 0.152: v52.83,42.55 52.83,41.88 LED2.1
  Bottom 0.152: v52.83,42.55 R44.1
N$13  (via drill 0.25)
  Top 0.152: v52.83,47.12 52.83,46.45 LED3.1
  Bottom 0.152: v52.83,47.12 R45.1
N$14  (via drill 0.25)
  Top 0.152: U0.4 32.79,34.56 32.51,34.29 32,34.29 31.75,34.04 v31.75,30.23 | 27.94,31.38 v27.94,30.23 27.94,31.5 | C2.2 R1.1
  Top 0.203: 27.94,31.38 R1.1 | R1.1 27.81,31.5 27.94,31.5
  Route15 0.152: v27.94,30.23 28.57,30.23 28.7,30.35 28.96,30.35 29.08,30.23 v31.75,30.23
  Bottom 0.152: C3.1 27.7,27.69 | 27.69,27.43 27.69,30.1 v27.94,30.23 27.7,30.21 C4.1
  Bottom 0.203: 27.83,27.69 27.7,27.69 27.56,27.69 27.56,27.56 27.69,27.43
N$15  (via drill 0.25)
  Top 0.152: U0.43 30.13,36.35 29.95,36.2 29.95,35.89 29.46,35.41 29.46,29.21 29.21,28.96 v28.83,28.96
  Route15 0.152: v28.83,28.96 26.8,28.96 v25.78,29.97
  Bottom 0.152: v25.78,29.97 25.78,29.08
  Bottom 0.203: R2.2 25.78,29.08 C3.2
N$16  (via drill 0.25)
  Top 0.152: U0.44 30.52,35.85 30.48,35.81 30.48,35.56 29.97,35.05 29.97,28.57 v28.83,27.43
  Route15 0.152: v28.83,27.43 26.67,27.43 v25.78,26.54
  Bottom 0.152: v25.78,26.54 25.78,27.54 25.77,27.55
  Bottom 0.203: R3.2 25.29,27.54 25.77,27.55 26.16,27.56 C4.2
N$17  (via drill 0.25)
  Top 0.152: 27.94,50.69 27.94,52.32 28.45,52.32 28.57,52.2 v28.7,52.2 29.97,52.2 | C11.2 R13.1 | U1.4 32.79,53.49 32.77,53.47 32.26,53.47 31.75,52.96 31.75,51.05 29.97,51.05 29.97,52.2 | U1.43 U1.44 30.01,54.9 29.97,54.86 29.97,52.2
  Top 0.203: 27.94,50.69 R13.1
N$18  (via drill 0.25)
  Top 0.152: v52.83,51.69 52.83,51.02 LED4.1
  Bottom 0.152: v52.83,51.69 R46.1
N$19  (via drill 0.25)
  Top 0.152: v52.83,56.26 52.83,55.59 LED5.1
  Bottom 0.152: v52.83,56.26 R47.1
N$20
  Top 0.152: C5.2 30.99,33.27 31.24,33.53 31.24,35.11 U0.1
N$21  (via drill 0.25)
  Route2 0.152: v49.02,72.64 49.28,72.64 49.78,72.14 49.78,53.59 49.28,53.09 49.28,52.58 49.78,52.07 49.78,29.34 v50.04,29.08
  Route15 0.152: v39.12,72.64 v49.02,72.64
  Bottom 0.152: R67.2 R66.2 R68.1 39,72.76 v39.12,72.64 | v50.04,29.08 50.55,29.08 50.8,29.34 50.8,30.02 M7.3
N$23  (via drill 0.25)
  Route2 0.152: v48.13,81.28 48.26,68.83 48.26,41.15 49.02,40.39 v49.02,32.03
  Route15 0.152: v31.88,81.79 32.26,81.28 v48.13,81.28
  Bottom 0.152: R69.1 R64.2 R65.2 32.02,81.93 v31.88,81.79 | v49.02,32.03 50.19,32.03 50.8,32.77 50.8,33.95 M6.3
N$24
  Top 0.152: U1.28 34.29,61.97 34.67,62.36 35.69,62.36 36.2,62.87 36.2,64.39 35.94,64.64 35.32,64.64 C13.1
N$25
  Top 0.152: U1.29 33.79,60.96 33.78,61.98 34.54,62.74 35.18,62.74 35.31,62.87 C13.2
N$26
  Top 0.152: 35.31,54.18 U1.9 U1.8 35.05,54.2 35.05,52.07 35.42,51.7 C14.1
N$27
  Top 0.152: C12.2 30.73,51.82 30.73,52.96 31.29,53.51 U1.1
N$28  (via drill 0.25)
  Top 0.152: LED8.N v23.11,68.07
  Bottom 0.152: v23.11,68.07 LED8.N
N$29  (via drill 0.25)
  Top 0.152: LED7.N v23.11,69.6
  Bottom 0.152: v23.11,69.6 LED7.N
N$30  (via drill 0.25)
  Top 0.152: LED6.N v23.11,71.12
  Bottom 0.152: v23.11,71.12 LED6.N
N$34
  Bottom 0.152: C32.2 48.27,18.91 48.51,18.67 49.41,18.67 U2.4
N$36  (via drill 0.25)
  Top 0.152: v52.83,40.51 52.83,41.18 LED2.3
  Bottom 0.152: v52.83,40.51 R40.1
N$42  (via drill 0.25)
  Top 0.152: v52.83,45.09 52.83,45.75 LED3.3
  Bottom 0.152: v52.83,45.09 R41.1
N$48
  Top 0.152: U0.28 34.29,42.92 34.67,43.31 35.56,43.31 36.2,43.94 36.2,45.34 35.94,45.59 35.32,45.59 C6.1
N$49
  Top 0.152: U0.29 33.79,42.93 34.54,43.69 35.18,43.69 35.31,43.81 C6.2
N$52
  Top 0.152: U0.8 U0.9 35.05,35.15 35.05,32.77 35.42,32.4 C7.1
N$56  (via drill 0.25)
  Top 0.152: v52.83,49.66 52.83,50.32 LED4.3
  Bottom 0.152: v52.83,49.66 R42.1
N$83  (via drill 0.25)
  Top 0.152: v52.83,54.23 52.83,54.9 LED5.3
  Bottom 0.152: v52.83,54.23 R43.1
PFET_GATE  (via drill 0.25)
  Route2 0.152: v44.96,64.01 v44.96,45.97
  Bottom 0.152: R11.2 R10.1 44.96,64.77 | M2.1 45.67,64.77 44.96,64.77 | 44.96,64.77 v44.96,64.01 | v44.96,45.97 45.47,45.97 45.72,46.23 45.72,46.78 M1.1
PG0  (via drill 0.25)
  Top 0.152: M3.2 55.37,43.69 TP3.TP1 55.63,41.66 55.02,41.18 LED2.4 | U0.14 38.07,36.35 38.35,36.07 38.35,34.8 37.08,33.27 | 37.08,33.27 R8.1 | 37.08,33.27 v37.34,33.53
  Route15 0.152: v37.34,33.53 39.75,33.53 39.88,33.66 40.51,33.66 41.15,34.29 52.58,34.29 56.52,30.35 58.29,30.35 59.31,31.37 59.31,39.75 TP3.TP1
PG1  (via drill 0.25)
  Top 0.152: TP4.TP1 55.63,46.23 55.15,45.75 LED3.4 53.85,45.75 53.85,45.09 53.09,44.32 53.09,43.94 52.83,43.69 M3.5 | U0.15 38.33,36.85 38.73,36.45 38.73,33.15 | 38.73,33.15 38.61,33.02 R9.1 | 38.73,33.15 40.01,33.15 v40.13,33.02
  Route15 0.152: v40.13,33.02 40.89,33.02 41.66,33.78 52.07,33.78 56.13,29.72 58.42,29.72 59.69,30.99 59.69,43.94 TP4.TP1
PG2  (via drill 0.25)
  Top 0.152: M4.2 55.37,52.83 TP5.TP1 55.63,50.8 55.02,50.32 LED4.4 | U1.14 37.51,55.37 38.23,55.37 38.86,54.74 R18.1 38.86,51.18 38.73,51.05 36.58,51.05 36.45,50.93 36.45,49.78 v36.2,49.53
  Route15 0.152: TP5.TP1 43.05,50.8 42.67,50.42 37.08,50.42 v36.2,49.53
PG3  (via drill 0.25)
  Top 0.152: TP6.TP1 55.63,55.37 55.15,54.9 LED5.4 54.1,54.9 54.1,54.48 53.09,53.47 53.09,53.09 52.83,52.83 M4.5 v50.04,52.83 | U1.15 38.59,55.9 40.39,54.1 | 40.39,54.1 R19.1 | 40.39,54.1 v41.66,54.1
  Route15 0.152: v41.66,54.1 48.77,54.1 v50.04,52.83
PGOOD0
  Top 0.203: J1.9 11.18,20.83 16.38,20.83 J2.9
  Bottom 0.152: J2.9 17.78,19.56 18.54,20.32 R51.1 R54.1
PGOOD1
  Top 0.203: J1.21 11.18,36.07 16.38,36.07 J2.21
  Bottom 0.152: R52.1 R55.1 18.54,35.56 17.78,34.8 J2.21
PGOOD2
  Top 0.203: J1.35 11.18,53.85 16.38,53.85 J2.35
  Bottom 0.152: J2.35 17.78,52.58 18.54,53.34 R56.1 R53.1
PGOOD3  (via drill 0.25)
  Top 0.203: J1.47 11.18,69.09 16.38,69.09 J2.47
  Route2 0.152: v11.18,4.32 11.18,66.55 J1.47
  Route15 0.152: J4.P$13 28.96,4.32 v11.18,4.32
  Bottom 0.152: J2.47 R57.1
PWRGD  (via drill 0.25)
  Top 0.152: v37.27,52.51 37.21,52.2 R20.1 37.27,51.9 v37.27,52.51 | U1.12 36.83,54.16 36.83,53.72 37.21,53.34 37.21,52.58 v37.27,52.51 | U0.12 36.79,34.59 v37.08,34.29
  Route2 0.152: v44.2,52.58 44.2,36.2 44.45,35.94 v44.45,35.56 44.45,35.18 44.2,34.92 v44.2,19.81
  Route15 0.152: v37.08,34.29 40.01,34.29 41.4,35.69 41.91,35.69 42.04,35.56 v44.45,35.56 | v44.2,52.58 43.43,53.34 38.23,53.34 v37.27,52.51 | v44.2,19.81 JP6.4
RESETB  (via drill 0.25)
  Top 0.152: v48.01,7.11 48.51,7.62 SW1.SW1 48.51,11.43 v50.04,12.95 | U1.16 39.36,56.4 v41.02,55.12 | 39.62,37.34 37.5,37.34 U0.16 39.61,37.35 39.62,37.34 | 39.62,37.34 v40.13,36.83
  Route2 0.152: J5.P$11 27.69,75.18 26.92,74.42 v26.92,65.28 26.92,63.25 27.18,62.99 27.18,45.21 27.69,44.7 27.69,42.67 27.18,42.16 v27.18,26.67 27.18,26.16 27.43,25.91 27.43,10.67 27.69,10.41 J4.P$11 | v41.02,55.12 41.02,54.99 40.89,54.86 40.89,38.86 v40.13,36.83 40.13,34.04 40.77,33.4 40.77,31.5 40.13,30.86 v40.13,26.8
  Route15 0.152: v48.01,7.11 29.21,7.11 J4.P$11 | v50.04,12.95 54.99,12.95 v55.75,13.72 | v23.11,65.28 v26.92,65.28 | v40.13,26.8 27.81,26.8 27.69,26.67 v27.18,26.67
  Bottom 0.152: JP6.6 C9.2 55.75,14.72 v55.75,13.72 | RPU3.R1_1 22.95,65.19 v23.11,65.28
RUN_CH0  (via drill 0.25)
  Top 0.152: U0.41 29.98,37.35 28.7,36.32 28.7,35.31 26.42,35.31 | 26.42,35.31 R6.1 | 26.42,35.31 v21.84,35.31
  Route2 0.152: v21.84,35.31 21.84,34.04 22.48,33.4 22.48,25.27 22.23,25.02 22.23,24.26 22.35,24.13 v22.35,23.75
  Route15 0.152: v22.35,23.75 20.7,23.75 20.45,23.5 16.51,23.5 J2.12
  Bottom 0.203: J1.12 8.64,23.37 13.84,23.37 J2.12
RUN_CH1
  Top 0.152: U0.40 29.98,37.85 29.72,37.85 29.46,37.34 28.57,36.83 27.94,36.83 | 27.94,36.83 R7.1 | 27.94,36.83 21.84,36.83 21.34,37.34 19.3,37.34 18.29,38.35 16.13,38.35 J2.24
  Bottom 0.203: J1.24 8.64,38.61 13.84,38.61 J2.24
RUN_CH2  (via drill 0.25)
  Top 0.152: U1.41 30.11,56.4 28.45,54.74 28.45,54.1 28.08,54.1 R16.1 27.83,53.1 27.81,53.09 22.61,53.09 v21.84,52.32
  Route15 0.152: v21.84,52.32 19.05,52.32 18.29,51.56 17.27,51.56 16.51,52.32 16.51,53.72 J2.38
  Bottom 0.203: J1.38 8.64,56.39 12.83,56.39 14.1,55.12 J2.38
RUN_CH3  (via drill 0.25)
  Top 0.152: U1.40 29.98,56.9 29.72,56.64 29.72,56.52 28.45,55.37 27.81,55.39 | 27.81,55.39 R17.1 | 27.81,55.39 27.81,56.01 27.69,56.13 v22.61,56.13
  Route2 0.152: v22.61,56.13 22.61,64.77 22.48,64.9 22.48,65.53 22.23,65.79 v22.23,69.6
  Route15 0.152: v22.23,69.6 20.32,69.6 18.54,71.37 16.13,71.37 J2.50
  Bottom 0.203: J1.50 8.64,71.63 13.84,71.63 J2.50
SCL  (via drill 0.25)
  Top 0.152: U0.21 38.07,39.85 38.15,39.93 38.61,39.93 v38.86,40.13 | v38.99,58.93 37.51,58.93 U1.21
  Route2 0.152: v38.86,40.13 38.86,40.77 38.99,40.89 38.99,41.4 38.86,41.53 38.86,44.45 38.94,44.53 38.94,44.88 38.86,44.96 38.86,45.47 38.79,45.54 38.79,45.9 38.86,45.97 38.86,48.13 38.99,48.26 v38.99,48.64 38.99,49.02 38.86,49.15 38.86,58.8 v38.99,58.93 38.99,59.82 39.12,59.94 v39.12,71.63
  Route15 0.152: v39.12,71.63 39.5,71.63 39.62,71.75 40.13,71.75 40.26,71.63 v49.02,71.63 | v38.86,40.13 40.39,40.13 41.66,38.86 55.37,38.86 TP1.TP1
  Bottom 0.152: v49.02,71.63 48.9,71.25 47.87,71.25 U3.2 | RPU1.R2_1 38.88,48.62 v38.99,48.64
SCL_IN  (via drill 0.25)
  Route2 0.152: J5.P$5 18.8,74.68 18.8,7.87 20.07,6.6 J4.P$5
  Route15 0.152: v21.08,73.15 21.84,72.39 27.69,72.39 28.19,71.88 37.08,71.88 38.99,69.98 48.51,69.98 v49.02,70.36 49.4,70.23 57.78,70.23 58.66,69.36 J3.4
  Bottom 0.152: R60.2 55.36,68.72 55.88,68.33 57.69,68.33 J3.4 | J5.P$5 20.07,74.17 v21.08,73.15 | U3.3 47.89,70.61 48.77,70.61 v49.02,70.36
SDA  (via drill 0.25)
  Top 0.152: U0.20 38.33,39.35 v38.35,39.37 | v39.75,58.42 39.37,58.42 39.24,58.29 38.61,58.29 38.48,58.42 37.51,58.42 U1.20
  Route2 0.152: v39.88,71.12 39.75,70.99 v39.75,58.42 39.37,58.04 39.37,49.15 39.62,48.9 39.62,48.39 39.37,48.13 v39.37,45.72 39.37,40.64 39.5,40.51 39.5,39.75 39.12,39.37 v38.35,39.37
  Route15 0.152: v38.35,39.37 37.85,38.86 37.85,38.1 38.35,37.59 40.39,37.59 40.89,37.08 40.89,36.32 53.34,36.32 TP2.TP1
  Bottom 0.152: v39.88,71.12 40.01,71.25 43.06,71.25 U3.7 | RPU1.R1_1 40.17,46.52 v39.37,45.72
SDA_IN  (via drill 0.25)
  Route2 0.152: J5.P$7 20.32,73.66 20.32,16.51 20.07,16.26 20.07,15.24 20.32,14.99 20.32,8.89 22.61,6.6 J4.P$7
  Route15 0.152: v22.61,73.15 27.43,73.15 28.19,72.39 37.08,72.39 38.99,70.48 40.01,70.48 40.13,70.61 v44.45,70.61 44.83,70.99 55.12,70.99 55.37,71.25 55.37,71.88 55.88,72.39 57.66,72.39 58.66,71.39 J3.2
  Bottom 0.152: J3.2 57.59,70.23 53.34,70.23 52.32,69.34 R59.2 | J5.P$7 v22.61,73.15 | U3.6 43.19,70.61 v44.45,70.61
SHARE_CLK  (via drill 0.25)
  Top 0.152: U1.13 37.49,54.21 v37.44,54.1 | U0.13 37.49,35.16 v37.47,35.05
  Route2 0.152: J5.P$14 31.37,77.34 31.37,75.06 30.73,74.42 30.73,71.63 30.61,71.5 30.61,68.58 30.73,68.45 v30.73,66.55 v30.66,54.1 v30.68,34.92 30.73,23.88 32,22.61 32,20.83 30.73,19.56 30.73,7.11 31.5,6.35 31.5,4.32 J4.P$14
  Route15 0.152: v37.44,54.1 v30.66,54.1 | v37.47,35.05 35.81,35.05 33.27,32.51 31.75,32.51 30.73,33.53 v30.68,34.92 | v24.51,66.04 28.45,66.04 29.08,66.67 29.72,66.67 29.84,66.55 v30.73,66.55
  Route15 0.203: JP6.5 56.64,15.75 56.64,13.72 55.12,12.19 54.61,12.19 46.74,4.32 31.5,4.32 J4.P$14
  Bottom 0.152: RPU3.R2_1 24.15,62.12 24.51,62.48 v24.51,66.04
SPARE4  (via drill 0.25)
  Route2 0.152: J4.P$19 37.85,6.86 38.61,7.62 38.61,19.81 39.37,20.57 39.37,22.35 43.69,26.67 43.69,52.07 43.43,52.32 43.43,52.83 43.69,53.09 v43.69,75.95
  Route15 0.152: v43.69,75.95 J5.P$19
TEMP_CH0
  Bottom 0.152: R4.2 19.16,18.27 18.54,18.29 16.38,18.29 J2.8
  Bottom 0.203: J1.8 8.64,18.29 13.84,18.29 J2.8
TEMP_CH1
  Bottom 0.152: R5.2 19.67,31.61 19.3,31.24 16.13,31.24 J2.20
  Bottom 0.203: J1.20 8.64,33.53 13.84,33.53 J2.20
TEMP_CH2
  Bottom 0.152: J2.34 15.11,50.16 16,51.05 18.29,51.05 19.18,50.16 R14.2
  Bottom 0.203: J1.34 8.64,51.31 13.84,51.31 J2.34
TEMP_CH3
  Bottom 0.152: R15.2 19.67,65.14 18.8,64.26 16.13,64.26 J2.46
  Bottom 0.203: J1.46 8.64,66.55 13.84,66.55 J2.46
USB_3.3V
  Route2 0.254: J4.P$1 12.32,8.26 12.32,73.28 J5.P$1
  Bottom 0.152: 44.7,73.24 44.7,73.49
  Bottom 0.203: M1.3 M2.3 47.69,67.24 | 47.69,67.24 47.75,67.31 52.21,67.31 R59.1 | 46.74,71.75 46.74,68.19 47.69,67.24 | J5.P$1 14.99,76.71 16.26,77.98 16.26,81.53 17.78,83.06 40.39,83.06 44.7,78.74 44.7,73.49 | C34.1 44.7,73.24 44.7,71.75 | 46.74,71.75 44.7,71.75 | 44.7,71.75 43.2,71.75 U3.8 | 46.74,71.75 47.73,71.75 U3.1
  Bottom 0.254: R59.1 R60.1 54.23,67.29 J3.5
USB_5V
  Bottom 0.203: R61.2 R62.2
  Bottom 0.254: J3.1 56.59,71.36 R62.2 | R61.2 52.31,71.37 51.31,71.37 50.2,72.48 U4.4 48.11,76.27 C35.1
VDD33_A  (via drill 0.25)
  Top 0.152: U0.6 U0.7 34.06,35.15 34.04,35.18 C8.1 34.04,32.26 34.8,32.26 34.8,29.97 v35.18,29.59 | R6.2 R7.2 28.81,34.66 v28.83,34.67
  Route2 0.152: v50.57,31.11 50.57,31.62 | v28.83,34.67 v28.83,29.72
  Route2 0.203: JP1.1 50.29,26.43 50.8,26.92 50.8,30.35 50.8,30.73 v50.57,31.11 50.57,31.62 v50.66,43.94
  Route15 0.152: JP2.1 JP3.1 46.28,43.94 v50.66,43.94 | v50.57,31.11 v50.56,31.11 50.04,31.11 49.91,30.99 38.86,30.99 37.47,29.59 v35.18,29.59 31.5,29.59 31.37,29.72 v28.83,29.72
  Bottom 0.152: U2.3 51.5,18.61 51.31,18.8 51.31,20.32 51.44,20.45 51.5,20.51 U2.1 | M1.2 46.59,48.15 46.74,48.01 46.74,46.23 46.23,45.72 JP3.1
  Bottom 0.203: R40.2 R44.2 v50.66,43.94 R41.2 R45.2 | JP1.1 50.32,26.38 51.31,25.4 51.31,20.7 51.5,20.51
  pour Top (no thermals): 33.66,35.56 34.42,35.56 34.42,32.13 33.66,32.13
VDD33_B  (via drill 0.25)
  Top 0.152: R17.2 R16.2 22.35,53.85 21.84,54.36 v20.95,54.36 | U1.6 U1.7 | C15.1 v34.04,52.58
  Top 0.203: v28.45,73.66 26.92,73.66 25.65,72.39 25.65,71.14 LED6.P LED7.P LED8.P
  Route2 0.203: v20.95,23.11 v20.95,36.58 v20.95,54.36 | v45.72,67.06 v45.72,74.55
  Route15 0.152: v28.45,73.66 32.77,73.66 33.27,73.41 34.8,73.41 35.31,73.66 38.86,73.66 v39.12,74.04 | JP4.1 JP5.1 | v50.55,61.72 46.02,61.72 JP5.1 | v45.72,67.06 45.97,66.8 JP5.1 | v34.04,52.58 34.04,49.28 35.56,47.75 49.91,47.75 v50.67,48.51
  Route15 0.203: v45.72,74.55 43.56,74.55 43.05,74.04 v39.12,74.04
  Bottom 0.152: R54.2 20.97,23.1 v20.95,23.11 | v20.95,36.58 20.95,35.58 R55.2 | R56.2 20.97,54.34 v20.95,54.36 21,54.4 RPU3.R4_2 RPU3.R3_2 RPU3.R2_2 RPU3.R1_2 21.08,63.1 21.08,63.5 22.48,64.9 22.48,65.53 20.95,67.06 20.95,67.44 R57.2 | R70.2 20.97,81.93 21.59,82.55 38.61,82.55 38.99,82.17 38.99,81.03 38.61,80.64 37.99,80.64 R69.2 38.62,80.63 39.12,80.14 v39.12,74.04 37.99,74.04 37.92,74.11 37.86,74.04 R68.2 | R47.2 50.66,61.61 v50.55,61.72 | M2.2 45.72,66.25 v45.72,67.06 | v50.67,48.51 50.67,49.64 R42.2
  Bottom 0.203: R43.2 R47.2 R46.2 R42.2 | R57.2 20.97,70.25 24.38,73.66 v28.45,73.66
  pour Top (no thermals): 33.66,54.61 34.42,54.61 34.42,51.44 33.66,51.44
VDDIO  (via drill 0.25)
  Top 0.152: R20.2 R18.2 R19.2 40.4,50.42 41.27,50.42 v42.16,51.31 | 35.81,41.27 35.81,41.08 U0.25 35.79,41.25 35.81,41.27 | U1.25 35.79,60.93 36.58,61.72 v37.34,61.72 | v40.13,31.75 39.48,31.1 R9.2 R8.2 v37.08,30.23 | 35.81,41.27 v35.81,41.91
  Route2 0.152: v37.34,61.72 37.9,61.16 37.9,54.59 37.97,54.48 37.97,48.39 37.85,48.26 37.85,44.96 37.77,44.88 37.77,44.53 37.85,44.45 v37.85,42.16 | v47.24,29.84 v47.24,33.02 | v35.81,41.91 35.81,38.61 36.07,38.35 36.07,37.85 35.81,37.59 35.81,34.54 35.05,33.78 35.05,32.26 v37.08,30.23
  Route15 0.152: v40.13,31.75 41.15,31.75 42.42,33.02 v47.24,33.02
  Bottom 0.152: RPU1.R3_2 RPU1.R4_2 42.12,51.27 v42.16,51.31 | RPU1.R1_2 42.05,47.66 R12.2 42.05,45.35 41.91,45.21 41.4,45.21 38.35,42.16 v37.85,42.16 37.47,42.55 36.2,42.55 35.81,42.16 v35.81,41.91 | M7.1 47.3,29.15 47.24,29.21 v47.24,29.84 | M6.1 48.62,33.02 v47.24,33.02 46.48,33.78 46.48,36.07 47.31,36.9 M5.1
  Bottom 0.203: RPU2.R1_2 RPU2.R2_2 43.65,29.68 43.69,29.46 45.85,29.46 C36.1 46.18,29.28 47.2,29.28 47.32,29.16 M7.1 48.68,27.6 48.13,27.05 48.18,25.48 JP1.2
  Bottom 0.254: RPU1.R3_2 RPU1.R2_2 RPU1.R1_2 | RPU2.R4_2 43.65,29.68 RPU2.R3_2 RPU2.R2_2
VIN  (via drill 0.25)
  Top 0.152: 33.27,35.14 U0.5 | 33.27,54.19 U1.5 33.29,53.35 v32.51,52.58
  Top 0.203: 33.27,54.19 33.27,53.34 v32.51,52.58 C10.1 | 33.27,35.14 33.27,34.04 v32.51,33.27 C1.1
  Route2 0.152: v32.51,52.58 32.51,56.13 32,56.64 32,57.66 32.51,58.17 32.51,66.29 v32.77,66.55
  Route15 0.152: v32.77,66.55 41.15,66.55 v41.4,66.29
  Bottom 0.152: v41.4,66.29 R11.1
  Bottom 0.254: J1.26 J1.25 J2.26 J2.25
  pour Route15 (isolate 0.203): 6.35,40.64 6.1,40.39 6.1,39.37 6.35,39.12 30.73,39.12 30.73,36.32 32,35.05 32,33.02 33.02,33.02 33.02,36.32 32,37.34 32,38.86 33.02,39.88 33.02,52.83 32,52.83 32,42.16 30.73,40.89 30.73,40.64 24.64,40.64 24.38,40.39 23.37,40.39 22.86,40.64
VIN_SNS  (via drill 0.25)
  Top 0.152: R1.2 26.53,30.85 26.29,30.61 24.26,30.61 24.13,30.48 v23.62,30.48 | R13.2 v23.37,50.8
  Route2 0.152: v21.08,15.75 22.99,17.65 22.99,20.57 22.86,20.7 22.86,22.86 23.62,23.62 v23.62,30.48 23.37,30.73 23.37,40.26 23.24,40.39 23.24,40.89 23.37,41.02 v23.37,50.8
  Route15 0.152: v21.08,15.75 16.38,15.75 J2.6
  Bottom 0.203: J1.6 8.64,15.75 13.84,15.75 J2.6
VIN_SNS_X
  Route2 0.152: J5.P$2 11.68,75.18 11.68,6.35 J4.P$2
VSM0
  Top 0.152: U0.33 31.79,42.89 30.99,43.69 29.46,43.69 29.34,43.81 R25.2 C21.1
VSM1
  Top 0.152: R27.2 C23.1 27.95,39.51 29.72,39.5 29.84,39.37 30.57,39.37 U0.37
VSM2
  Top 0.152: U1.33 31.79,62.07 31.24,62.61 30.1,62.61 29.97,62.74 29.46,62.74 29.48,63.37 R29.2 C25.1
VSM3
  Top 0.152: R31.2 C27.1 28.59,58.05 28.96,58.42 30.57,58.42 U1.37
VSNSM_CH0  (via drill 0.25)
  Top 0.152: R25.1 v27.05,44.45
  Top 0.203: J1.1 11.18,10.67 16.38,10.67 J2.1
  Route2 0.152: v1.14,45.34 1.14,44.83 1.02,44.7 1.02,26.92 1.78,26.16 1.78,9.4 3.05,8.13 8.64,8.13 J1.1
  Route15 0.152: v27.05,44.45 20.32,44.45 18.8,45.97 2.29,45.97 1.65,45.34 v1.14,45.34
VSNSM_CH1  (via drill 0.25)
  Top 0.152: R27.1 24.4,37.58 v22.73,37.59
  Top 0.203: J1.13 11.18,25.91 16.38,25.91 J2.13
  Route2 0.152: v22.73,37.59 22.73,33.91 22.86,33.78 v22.86,24.64
  Route15 0.152: v22.86,24.64 J2.13
VSNSM_CH2  (via drill 0.25)
  Top 0.152: R29.1 26.92,63.5 26.42,64.01 v25.78,64.01
  Top 0.203: J1.27 11.18,43.69 16.38,43.69 J2.27
  Route2 0.152: v13.21,63.75 v13.21,42.16
  Route15 0.152: v25.78,64.01 25.27,64.01 25.02,63.75 v13.21,63.75 | v13.21,42.16 13.97,41.4 16.64,41.4 J2.27
VSNSM_CH3  (via drill 0.25)
  Top 0.152: R31.1 25.8,56.75 25.15,57.4 v24.51,57.4
  Top 0.203: J1.39 11.18,58.93 16.38,58.93 J2.39
  Route15 0.152: v24.51,57.4 17.91,57.4 J2.39
VSNSP_CH0  (via drill 0.25)
  Top 0.152: R24.1 30.1,44.45 30.1,46.99 29.08,46.99 v28.7,47.24
  Route2 0.152: v1.65,46.48 1.65,46.1 2.29,45.47 2.29,42.8 2.16,42.67 2.16,42.16 2.29,42.04 2.29,10.16 3.05,9.4 J1.2
  Route15 0.152: v28.7,47.24 19.3,47.24 18.54,46.48 v1.65,46.48
  Bottom 0.203: J1.2 8.64,10.67 13.84,10.67 J2.2
VSNSP_CH1  (via drill 0.25)
  Top 0.152: R26.1 24.53,41.54 v24.51,41.53
  Route2 0.152: v3.56,41.4 3.56,29.46 3.81,29.21 v3.81,24.64
  Route15 0.152: v24.51,41.53 18.67,41.53 18.16,41.02 4.45,41.02 4.06,41.4 v3.56,41.4 | v3.81,24.64 J1.14
  Bottom 0.203: J1.14 8.64,25.91 13.84,25.91 J2.14
VSNSP_CH2  (via drill 0.25)
  Top 0.152: R28.1 29.97,63.5 29.97,65.66 v29.46,66.04
  Route2 0.152: v1.78,63.75 1.78,47.5 2.29,46.99 2.29,46.48 2.79,45.97 v2.79,42.42
  Route15 0.152: v29.46,66.04 29.46,64.26 26.42,64.26 26.04,64.64 25.4,64.64 25.02,64.26 13.59,64.26 13.46,64.39 12.95,64.39 12.83,64.26 2.79,64.26 2.29,63.75 v1.78,63.75 | v2.79,42.42 J1.28
  Bottom 0.203: J1.28 8.64,43.69 13.84,43.69 J2.28
VSNSP_CH3  (via drill 0.25)
  Top 0.152: R30.1 25.64,60.72 25.4,60.96 v24.51,60.96
  Route15 0.152: v24.51,60.96 20.07,60.96 18.29,59.18 16.64,59.18 J2.40
  Bottom 0.203: J1.40 8.64,58.93 13.84,58.93 J2.40
VSP0
  Top 0.152: U0.32 32.29,43.15 32,43.43 32,44.44 R24.2 C20.1
VSP1
  Top 0.152: R26.2 C22.1 29.73,40.24 30.1,39.88 30.56,39.88 U0.36
VSP2
  Top 0.152: U1.32 32.29,62.2 32,62.48 32,63.48 R28.2 C24.1
VSP3
  Top 0.152: R30.2 C26.1 28.72,59.42 29.21,58.93 30.56,58.93 U1.36

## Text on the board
tPlace: INSTALL CONNECTORS | ON TOP SIDE | (408) 432-1900 | www.linear.com | GND | F | E | M | A | L | E | DEMO CIRCUIT 2675A | 50 | ALERT | FAULTB0 | FAULTB1 | 47 | 46 | ASEL1 | ASEL0 | 43 | 42 | LTC2972 | HIGH | FLOAT | 39 | PG3 | 38 | LOW | 35 | PG2 | 34 | PG1 | 31 | 30 | ASEL1 | ASEL0 | HIGH | PG0 | 27 | LTC2972 | FLOAT | 26 | LOW | SCL | 23 | 22 | SDA | 19 | 18 | VDDIO | ALRT | 15 | Dual CH Power | System Manager | 3.3V | 14 | FLT0 | CTRL0 | CTRL1 | CTRL2 | CTRL3 | 1.8V | FLT1 | 11 | 10 | PWRGD | RUN | RUN | RUN | RUN | SCLK | 7 | RESET | 6 | RST | AUX | 3 | 2 | OFF | OFF | OFF | OFF | M | A | L | E | GND
bPlace: LTC CONFIDENTIAL | FOR CUSTOMER USE ONLY | Rev 1 / mtp
d_FabDrawing: 3.400" | DRILL TABLE | 0.00" | 0.00" | 2.40"
DrillLegend: LAYER-STACK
